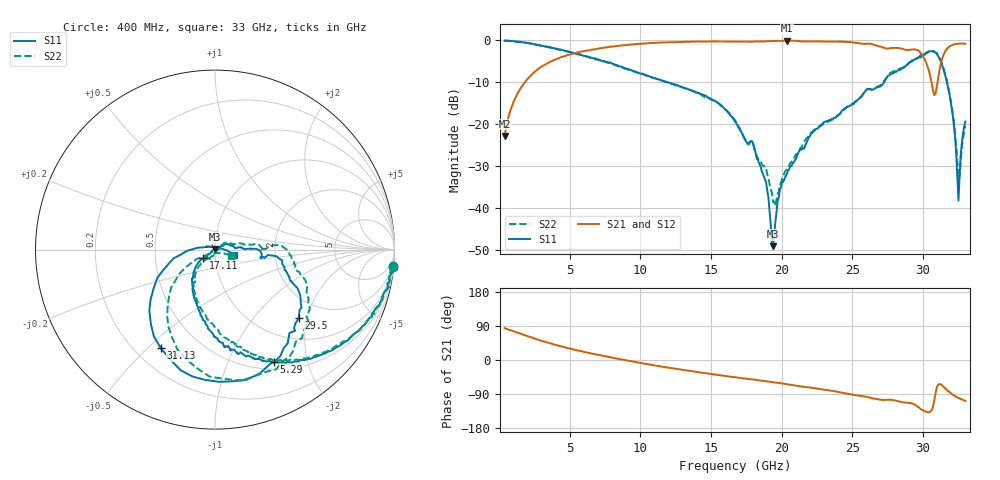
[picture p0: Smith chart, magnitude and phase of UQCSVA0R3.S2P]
!  Part Number  UQCSVA0R3  Mounting Orientation: Horizontal
!  Description: Ultra Low ESR Microwave capacitors
!  Application: Coupling, Bypass, Tuning, DC Block
!  Filters, Matching
# GHZ S DB R 50
! Freq  |S11|  S11 Ph  |S21|  S21 Ph  |S12|  S12 Ph  |S22|  S22 Ph
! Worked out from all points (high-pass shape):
!   401 points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, 400 MHz to 33 GHz, reference 50 ohm
!   highest |S21| = -0.06 dB at 20.37 GHz (marker M1); lowest = -22.8 dB at 400 MHz (marker M2)
!   |S21| within 3 dB of the highest: 5.317 GHz to 29.84 GHz (24.52 GHz wide, 140 % of centre); 31.5 GHz to end of sweep
!   lowest |S11| = -49.2 dB at 19.39 GHz (marker M3), VSWR 1.01, Z = 49.9 + j0.33 ohm
!   |S11| at or under -10 dB: 11.88 GHz to 27.24 GHz (15.36 GHz wide, 78.5 % of centre); 31.7 GHz to end of sweep
!   |S22| runs from -39.6 to 0.0 dB; largest |S21 - S12| = 0.016
!   S11 on the Smith chart (normalised r, x): 400 MHz: 1, -22; 5.29 GHz: 0.59, -1.49; 17.11 GHz: 0.87, -0.08; 29.5 GHz: 1.48, -1.77; 31.13 GHz: 0.30, -0.55; 33 GHz: 1.23, -0.07
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0.4  -0.05 -5.2  -22.84 84.3  -22.83 84.2  -0.03 -5.7
1.134  -0.23 -13.9  -13.94 74.7  -13.96 73.6  -0.27 -16.8
2.112  -0.67 -27.5  -8.90 62.1  -8.93 61.1  -0.71 -28.6
5.29  -2.98 -62.3  -3.08 27.6  -3.03 28.2  -2.96 -60.9
5.861  -3.54 -67.4  -2.67 22.9  -2.62 23.2  -3.49 -65.3
11.321  -9.36 -106.2  -0.53 -16.2  -0.50 -16.2  -9.37 -103.0
16.7  -19.40 -142.9  -0.27 -45.8  -0.28 -45.7  -19.05 -135.0
17.108  -21.76 -144.0  -0.26 -47.6  -0.28 -47.5  -21.69 -134.3
17.923  -24.12 -140.4  -0.30 -51.0  -0.32 -50.7  -24.29 -117.9
18.738  -32.54 -143.3  -0.23 -55.1  -0.21 -54.8  -29.96 -96.1
19.39  -49.20 107.3  -0.13 -58.5  -0.11 -58.2  -38.66 -70.0
19.879  -35.64 31.1  -0.11 -61.0  -0.09 -60.7  -34.46 2.1
20.368  -31.96 25.5  -0.06 -63.9  -0.04 -63.5  -30.95 14.7
22.161  -22.19 21.5  -0.21 -73.5  -0.18 -73.3  -21.91 28.2
27.621  -8.34 -11.9  -1.90 -104.9  -1.89 -104.7  -7.94 -0.1
29.496  -4.39 -39.4  -2.20 -119.6  -2.13 -119.9  -4.46 -29.7
30.148  -3.15 -58.5  -4.75 -135.6  -4.82 -135.3  -3.32 -48.6
30.8  -2.76 -94.4  -13.07 -106.7  -12.83 -106.3  -2.66 -81.1
31.126  -4.05 -118.7  -7.99 -63.6  -7.91 -64.4  -3.99 -104.6
31.941  -14.26 -171.6  -1.31 -87.0  -1.30 -87.1  -14.02 -148.3
32.511  -38.31 68.6  -0.80 -100.2  -0.79 -100.4  -33.24 -102.5
33  -19.37 -15.6  -0.79 -107.8  -0.79 -107.9  -20.39 -21.6
